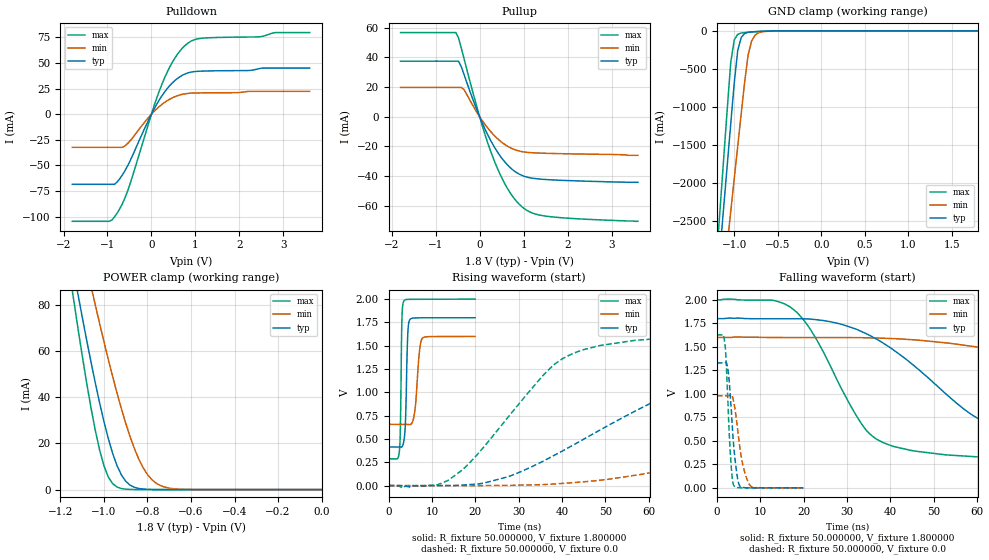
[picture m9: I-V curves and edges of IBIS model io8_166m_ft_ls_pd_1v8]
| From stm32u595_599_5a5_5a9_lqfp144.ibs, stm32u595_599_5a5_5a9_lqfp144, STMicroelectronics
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|   Model io8_166m_ft_ls_pd_1v8
[Model]  io8_166m_ft_ls_pd_1v8
Model_type I/O
Polarity   Non-Inverting
Enable   Active-Low
Vinl =   0.540000V
Vinh =   1.260000V
Vmeas =  0.900000V
Cref =   50.000000pF
Rref =   100.000000M
Vref =   0.0V
C_comp   3.358100pF   3.352600pF   3.400200pF
[Temperature Range]   25.000000   0.140000k   -40.000000
[Pullup Reference]   1.800000V   1.600000V   2.000000V
[Pulldown Reference]   0.0V   0.0V   0.0V
[POWER Clamp Reference]   1.800000V   1.600000V   2.000000V
[GND Clamp Reference]   0.0V   0.0V   0.0V
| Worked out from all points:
|   slope of the pulldown table from 0 to 0.27 V, typ, clamps not added: 13.6 ohm
|   slope of the pullup table from 0 to 0.27 V, typ, clamps not added: 15.9 ohm
|   GND clamp passes 1 mA (typ) near -0.50 V on its own axis
|   POWER clamp passes 1 mA (typ) near -0.86 V on its own axis
|   rising waveform, R_fixture 50.000000, V_fixture 1.800000: 20-80 % time 442ps typ, 899ps min, 292ps max; typ from 0.414 V to 1.8 V
|   rising waveform, R_fixture 50.000000, V_fixture 0.0: 20-80 % time 34.1ns typ, 74.8ns min, 18ns max; typ from 0 V to 1.33 V
|   falling waveform, R_fixture 50.000000, V_fixture 1.800000: 20-80 % time 23.4ns typ, 59.3ns min, 12.2ns max; typ from 1.8 V to 0.414 V
|   falling waveform, R_fixture 50.000000, V_fixture 0.0: 20-80 % time 1.31ns typ, 1.9ns min, 974ps max; typ from 1.33 V to 0 V
[Pulldown]
|Voltage   I(typ)   I(min)   I(max)
-1.8V     -68.38mA   -32.32mA   -104.4mA
-960mV    -68.38mA   -32.32mA   -104.4mA
-780mV    -66.08mA   -32.32mA   -96.43mA
-660mV    -59.2mA    -32.31mA   -87.22mA
-540mV    -50.22mA   -28.51mA   -74.66mA
0V        -10fA      -200fA     0A
240mV     18.04mA    9.6mA      29.42mA
480mV     30.68mA    16.02mA    50.95mA
780mV     39.48mA    19.99mA    67.56mA
1.14V     41.99mA    20.78mA    74.01mA
2.82V     44.93mA    22.28mA    79.57mA
3.6V      44.93mA    22.28mA    79.57mA
[Pullup]
|Voltage   I(typ)   I(min)   I(max)
-1.8V     37.48mA    19.76mA    56.76mA
-540mV    37.48mA    19.76mA    56.76mA
-480mV    37.48mA    19.76mA    53.06mA
-360mV    28.94mA    18.48mA    39.74mA
0V        0A         0A         0A
300mV     -18.63mA   -11.6mA    -27.18mA
600mV     -31.41mA   -19.24mA   -46.67mA
780mV     -36.41mA   -22mA      -54.89mA
960mV     -39.54mA   -23.52mA   -60.64mA
1.2V      -41.44mA   -24.28mA   -64.93mA
1.56V     -42.42mA   -24.69mA   -67.24mA
3.6V      -44.2mA    -26mA      -70.5mA
[GND_clamp]
|Voltage   I(typ)   I(min)   I(max)
-1.8V     -9.908A    -9.683A    -9.994A
-1.2V     -3.383A    -4.084A    -2.934A
-1.16V    -2.841A    -3.655A    -2.294A
-1.12V    -2.299A    -3.226A    -1.656A
-1.04V    -1.218A    -2.369A    -414.2mA
-1V       -684.7mA   -1.941A    -119.2mA
-960mV    -257.2mA   -1.514A    -45.67mA
-920mV    -87.04mA   -1.089A    -28.94mA
-840mV    -19.36mA   -312.8mA   -18.98mA
-800mV    -13.56mA   -132.4mA   -15.51mA
-720mV    -8.053mA   -25.67mA   -9.505mA
1.8V      45.71uA    33.32uA    56.11uA
[POWER_clamp]
|Voltage   I(typ)   I(min)   I(max)
-1.8V     470.8mA    433.7mA    554.6mA
-1.14V    95.25mA    122.7mA    82.82mA
-1.12V    84.97mA    114mA      70.27mA
-1.06V    55.51mA    88.42mA    35.67mA
-1.04V    46.34mA    80.15mA    25.76mA
-1V       29.51mA    64.13mA    10.3mA
-940mV    10.39mA    41.86mA    1.109mA
-900mV    3.624mA    28.77mA    182.8uA
-840mV    490.7uA    13.24mA    11.35uA
-800mV    116.8uA    6.532mA    1.77uA
-740mV    13.2uA     1.724mA    109.3nA
0V        0A         18.75nA    0A
[Ramp]
| variable   typ   min   max
dV/dt_r  0.79740/34.07846n   0.58727/74.68967n   0.97632/17.98179n
dV/dt_f  0.83143/23.37608n   0.56491/59.20743n   1.02745/12.18749n
R_load = 50.000000
[Rising Waveform]
R_fixture= 50.000000
V_fixture= 1.800000
V_fixture_min= 1.600000
V_fixture_max= 2.000000
|time   V(typ)   V(min)   V(max)
0s        413.8mV    656.4mV    287.1mV
2.482ns   413.5mV    656.4mV    372.4mV
2.723ns   412.6mV    656.4mV    660.8mV
3.083ns   416.1mV    656.4mV    1.815V
3.483ns   470.5mV    656.4mV    1.979V
3.924ns   738.6mV    656.3mV    1.994V
4.404ns   1.615V     655.3mV    1.997V
4.885ns   1.779V     654mV      1.997V
7.688ns   1.799V     1.575V     1.998V
19.94ns   1.8V       1.599V     2V
[Rising Waveform]
R_fixture= 50.000000
V_fixture= 0.0
V_fixture_min= 0.0
V_fixture_max= 0.0
|time   V(typ)   V(min)   V(max)
0s        1.796nV    144.1nV    1.167nV
13.61ns   -219.1uV   -198.5uV   52.92mV
27.23ns   90.85mV    1.549mV    715.5mV
38.44ns   330.6mV    17.73mV    1.307V
56.86ns   798.9mV    110.5mV    1.557V
72.07ns   1.096V     237.2mV    1.601V
88.09ns   1.222V     384mV      1.618V
128.9ns   1.308V     710mV      1.626V
169ns     1.323V     877.7mV    1.627V
398.8ns   1.329V     979.8mV    1.627V
[Falling Waveform]
R_fixture= 50.000000
V_fixture= 1.800000
V_fixture_min= 1.600000
V_fixture_max= 2.000000
|time   V(typ)   V(min)   V(max)
0s        1.8V       1.599V     2V
16.82ns   1.798V     1.598V     1.926V
21.62ns   1.795V     1.598V     1.681V
35.24ns   1.622V     1.595V     574.5mV
52.85ns   998.3mV    1.542V     350.6mV
61.66ns   704.4mV    1.486V     325.1mV
72.87ns   567.4mV    1.388V     308.6mV
115.3ns   447.7mV    926.1mV    290.1mV
151.4ns   425.2mV    772.1mV    287.8mV
398.8ns   413.8mV    656.4mV    287.1mV
[Falling Waveform]
R_fixture= 50.000000
V_fixture= 0.0
V_fixture_min= 0.0
V_fixture_max= 0.0
|time   V(typ)   V(min)   V(max)
0s        1.329V     979.8mV    1.627V
1.842ns   1.33V      979.8mV    1.537V
2.162ns   1.334V     979.8mV    1.338V
2.723ns   1.197V     979.6mV    719.3mV
3.363ns   810.1mV    987.5mV    197.7mV
3.924ns   427.7mV    907.4mV    25.42mV
5.165ns   31.16mV    480.4mV    1.252mV
6.286ns   2.662mV    190.9mV    59.67uV
7.728ns   466.5uV    21.77mV    -104.4uV
19.94ns   1.796nV    144.1nV    1.167nV
